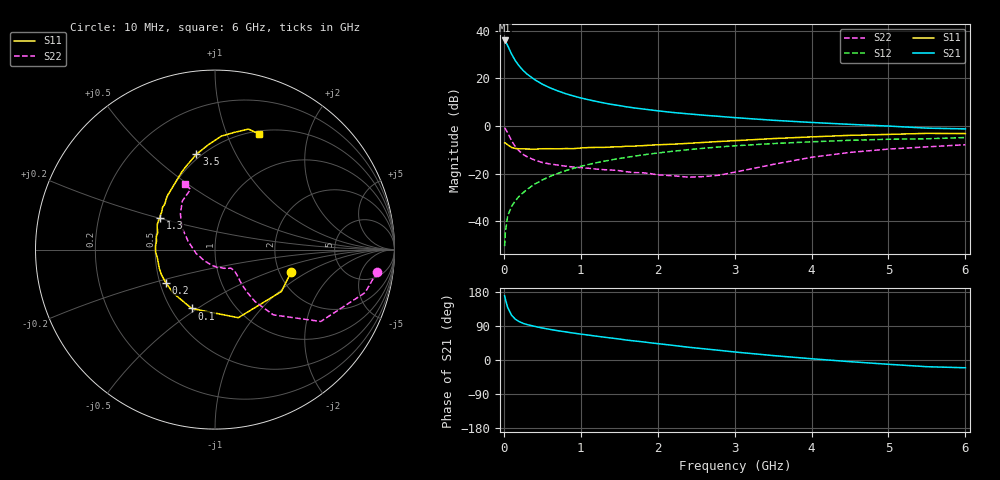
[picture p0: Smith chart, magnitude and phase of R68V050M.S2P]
! SIEMENS Small Signal Semiconductors
! BFR193
! Si NPN RF Bipolar Junction Transistor in SOT23
! VCE = 8 V  IC = 50 mA
! Common Emitter S-Parameters:  May  1996
# GHz  S  MA  R  50
!  f  S11  S21  S12  S22
! GHz  MAG  ANG  MAG  ANG  MAG  ANG  MAG  ANG
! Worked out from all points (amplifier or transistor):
!   36 points, 10 MHz to 6 GHz, reference 50 ohm
!   highest |S21| = 35.8 dB at 10 MHz (marker M1)
!   |S21| within 3 dB of that: start of sweep to 61.91 MHz
!   unconditionally stable (mu >= 1): 439.8 MHz to 2.105 GHz
!   at 250 MHz: K = 0.93, MSG = 25.7 dB, |S12| = -28.1 dB
!   at 1.4 GHz: K = 1.02, MAG = 10.7 dB, |S12| = -14.2 dB
!   at 6 GHz: K = 0.95, MSG = 1.8 dB, |S12| = -4.9 dB
!   S11 on the Smith chart (normalised r, x): 10 MHz: 2.32, -0.72; 100 MHz: 0.63, -0.47; 200 MHz: 0.54, -0.22; 1.3 GHz: 0.50, +0.20; 3.5 GHz: 0.47, +0.71; 6 GHz: 0.53, +1.31
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0.01  0.4425 -16.4  61.86 169.6  0.003 80.1  0.9117 -7.8
0.02  0.4373 -32.3  59.38 160.3  0.0059 77.4  0.8699 -16.0
0.05  0.4012 -71.1  48.23 138.5  0.0129 69.1  0.7124 -34.2
0.1  0.3529 -111.6  32.17 118.3  0.0204 67.2  0.4879 -48.2
0.15  0.3359 -133.7  23.18 107.6  0.0269 67.2  0.3652 -52.4
0.2  0.3303 -146.1  18 101.3  0.0336 69.3  0.2965 -53.0
0.25  0.3298 -155.0  14.57 96.8  0.0395 70.6  0.2521 -52.5
0.3  0.3275 -161.3  12.26 93.6  0.0463 72.4  0.2258 -51.5
0.4  0.3244 -171.5  9.341 88.8  0.0599 72.8  0.1917 -49.5
0.5  0.3312 -177.9  7.487 84.5  0.0732 73.2  0.1704 -48.0
0.6  0.3319 176.7  6.283 80.8  0.0873 72.6  0.1587 -47.7
0.7  0.3294 172.1  5.423 77.3  0.1006 72.0  0.1508 -48.1
0.8  0.3343 167.7  4.755 74.3  0.1142 70.7  0.1431 -48.8
1.1  0.3512 156.8  3.536 65.7  0.155 67.4  0.1293 -53.8
1.3  0.3535 150.3  3.025 60.3  0.1813 64.6  0.1207 -58.2
1.7  0.3771 138.0  2.372 50.2  0.2322 59.1  0.1048 -72.3
2.2  0.413 126.5  1.909 38.6  0.2941 51.7  0.09 -101.1
2.8  0.4708 113.1  1.582 25.5  0.3612 42.5  0.0924 -154.0
3.5  0.5416 101.0  1.311 11.7  0.4251 31.6  0.1556 163.2
4.5  0.6333 86.8  1.076 -4.4  0.498 17.7  0.2777 134.0
5.5  0.6967 74.5  0.896 -17.7  0.5364 4.1  0.3626 112.1
6  0.6895 69.1  0.864 -20.5  0.5694 0.4  0.4024 114.6
